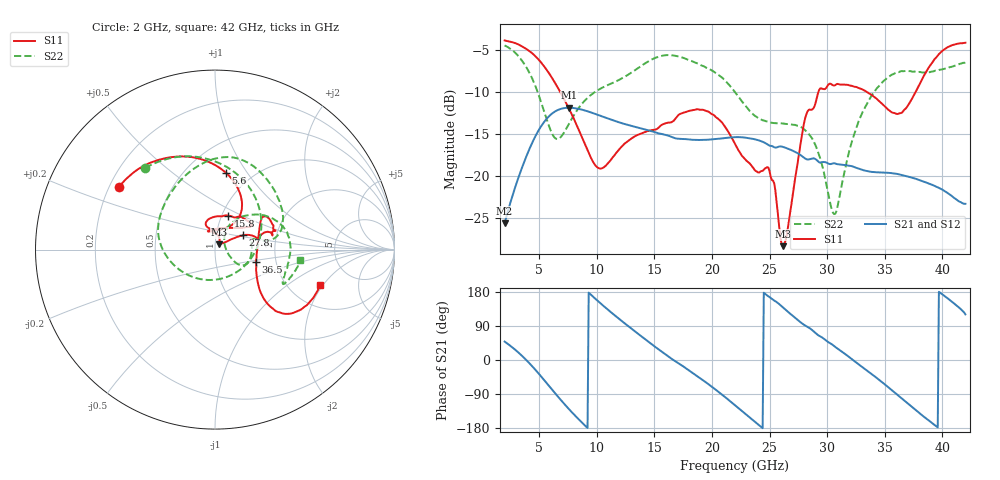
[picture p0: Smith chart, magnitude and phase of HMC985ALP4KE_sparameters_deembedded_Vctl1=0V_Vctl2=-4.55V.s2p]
!s2p File: Measurements: S11, S21, S12, S22
# GHz S dB R 50.0
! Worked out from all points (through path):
!   401 points, 2 GHz to 42 GHz, reference 50 ohm
!   highest |S21| = -11.89 dB at 7.6 GHz (marker M1); lowest = -25.7 dB at 2 GHz (marker M2)
!   lowest |S11| = -28.4 dB at 26.2 GHz (marker M3), VSWR 1.08, Z = 52.3 + j3.17 ohm
!   |S11| at or under -10 dB: 6.82 GHz to 29.25 GHz (22.43 GHz wide, 124 % of centre); 33.42 GHz to 37.69 GHz (4.269 GHz wide, 12 % of centre)
!   |S22| runs from -24.6 to -4.5 dB; largest |S21 - S12| = 0.00023
!   S11 on the Smith chart (normalised r, x): 2 GHz: 0.24, +0.28; 5.6 GHz: 0.76, +0.80; 15.8 GHz: 1.07, +0.42; 27.8 GHz: 1.34, +0.22; 36.5 GHz: 1.57, -0.23; 42 GHz: 2.94, -1.89
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2  -3.88 147.0  -25.66 48.6  -25.67 48.6  -4.47 130.5
3.6  -4.66 120.3  -18.70 8.4  -18.70 8.4  -6.47 84.9
4.7  -5.80 99.5  -15.21 -26.8  -15.22 -26.8  -9.41 43.4
5.6  -7.29 81.9  -13.29 -59.0  -13.30 -59.1  -13.05 -3.7
6.5  -9.22 66.5  -12.25 -92.0  -12.25 -92.0  -15.61 -68.9
7.6  -12.04 54.8  -11.89 -130.1  -11.90 -130.1  -13.77 -135.7
8.7  -15.38 55.1  -12.12 -164.7  -12.12 -164.7  -11.45 -170.2
10.4  -19.13 89.6  -12.89 147.5  -12.90 147.5  -9.57 162.5
15.4  -14.23 75.7  -14.97 27.5  -14.97 27.5  -5.80 87.1
15.8  -13.83 68.7  -15.07 18.6  -15.07 18.6  -5.67 82.1
19.4  -12.23 33.3  -15.72 -57.2  -15.72 -57.3  -7.05 35.1
22  -16.18 51.1  -15.40 -119.4  -15.41 -119.4  -10.04 9.9
24.9  -19.04 104.8  -16.34 167.9  -16.34 167.9  -13.58 13.3
26.2  -28.38 52.7  -16.57 137.5  -16.58 137.5  -13.78 -2.4
27.8  -15.23 27.3  -17.64 97.0  -17.64 97.0  -14.24 -24.4
28.7  -12.10 12.6  -17.93 78.9  -17.94 78.9  -15.56 -31.4
30.7  -9.21 20.8  -18.53 34.6  -18.53 34.6  -24.53 22.7
32.8  -9.59 33.9  -19.19 -13.0  -19.19 -13.0  -13.28 53.4
35.4  -12.22 11.8  -19.66 -74.2  -19.66 -74.2  -8.17 21.5
36.5  -12.47 -16.7  -19.91 -102.0  -19.91 -102.1  -7.54 7.4
39.5  -5.86 -43.8  -21.30 -175.5  -21.31 -175.5  -7.46 -26.4
42  -4.15 -18.6  -23.34 120.5  -23.34 120.4  -6.47 -7.2
